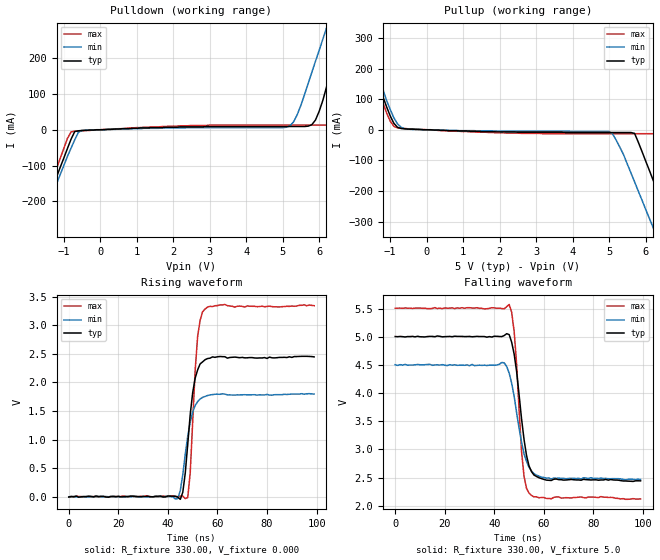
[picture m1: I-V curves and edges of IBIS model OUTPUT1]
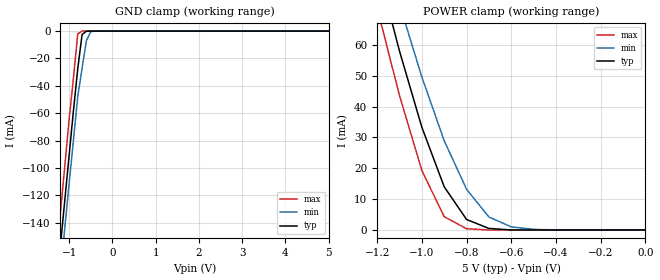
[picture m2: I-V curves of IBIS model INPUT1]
| IBIS file 8581nb5v.ibs
[IBIS ver]   2.1
[File name]   8581nb5v.ibs
[File Rev]   1.0
[Date]   July 4, 2003
[Source]   This file orginated at SEIKO EPSON QD Div.
   This file is for 5.0V CMOS parts.
[Copyright]   Copyright SEIKO EPSON Corp. 2003
|   Component RX-8581NB
[Component]   RX-8581NB
[Manufacturer]   SEIKO EPSON
[Package]
| variable   typ   min   max
R_pkg   87m   NA   NA
L_pkg   10nH   NA   NA
C_pkg   206fF   NA   NA
[Pin]  signal_name   model_name   R_pin   L_pin   C_pin
|1   /INT
2   GND   GND
|3   (VDD)
|4   NC
|5   SDA
|6   SCL
7   FOUT   OUTPUT1
8   VDD   POWER
9   FOE   INPUT1
| Models and submodels in the file (2): OUTPUT1 (Output), INPUT1 (Input)
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|10   NC
|11   NC
|12   NC
|13   NC
|14   NC
|15   NC
|16   NC
|17   NC
|18   NC
|19   NC
|20   NC
|21   NC
|22   NC
|   Model OUTPUT
[Model]   OUTPUT1
Model_type   Output
Polarity   Non-Inverting
Enable   Active-High
Vmeas =   1.50V
C_comp   1.69pF   1.32pF   1.96pF
[Temperature Range]   25.00   85.00   -40.000
[Voltage Range]   5.0V   4.5V   5.5V
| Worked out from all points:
|   slope of the pulldown table from 0 to 0.75 V, typ, clamps not added: 250 ohm
|   slope of the pullup table from 0 to 0.75 V, typ, clamps not added: 250 ohm
|   rising waveform, R_fixture 330.00, V_fixture 0.000: 20-80 % time 3.39ns typ, 3.85ns min, 2.5ns max; typ from -0.005 V to 2.45 V
|   falling waveform, R_fixture 330.00, V_fixture 5.0: 20-80 % time 4.13ns typ, 5.01ns min, 2.91ns max; typ from 5.01 V to 2.44 V
[Pulldown]
| voltage   I(typ)   I(min)   I(max)
-5V       -1.155A    -1.128A    -1.18A
-2V       -348mA     -357mA     -334mA
-1.5V     -213mA     -228mA     -193mA
-800mV    -26mA      -51mA      -6mA
-500mV    -2mA       -2mA       -3mA
5.2V      9mA        11mA       13mA
5.9V      27mA       191mA      13mA
6.3V      155mA      313mA      13mA
6.7V      303mA      436mA      97mA
7V        414mA      528mA      200mA
7.5V      598mA      681mA      372mA
10V       1.522A     1.447A     1.231A
[Pullup]
| voltage   I(typ)   I(min)   I(max)
-5V       1.467A     1.5A       1.488A
-2V       393mA      420mA      378mA
-1.5V     214mA      240mA      193mA
-1V       45mA       66mA       28mA
-700mV    4mA        8mA        5mA
5V        -9mA       -6mA       -13mA
5.3V      -9mA       -58mA      -13mA
5.7V      -12mA      -170mA     -13mA
6.3V      -192mA     -347mA     -15mA
6.8V      -345mA     -494mA     -156mA
7.5V      -558mA     -700mA     -354mA
10V       -1.321A    -1.435A    -1.062A
[Ramp]
| variable   typ   min   max
dV/dt_r 1.08/2.1n   0.88/2.7n   0.74/1n
dV/dt_f 0.6/1.8n   0.67/2.7n   1.04/1.7n
R_load = 330.00
[Rising Waveform]
R_fixture = 330.00
V_fixture = 0.000
| time   V(typ)   V(min)   V(max)
0s        -5mV       -1mV       -3mV
44ns      -8mV       -31mV      1mV
46ns      78mV       388mV      12mV
48ns      920mV      1.061V     -14mV
49ns      1.439V     1.304V     420mV
51ns      2.076V     1.597V     2.218V
52ns      2.221V     1.664V     2.81V
54ns      2.36V      1.739V     3.238V
63ns      2.45V      1.796V     3.364V
99ns      2.447V     1.796V     3.343V
[Falling Waveform]
R_fixture = 330.00
V_fixture = 5.0
V_fixture_min = 4.5
V_fixture_max = 5.5
| time   V(typ)   V(min)   V(max)
0s        5.006V     4.505V     5.509V
43ns      5.005V     4.545V     5.504V
46ns      5.04V      4.356V     5.575V
48ns      4.694V     3.945V     5.095V
49ns      4.383V     3.653V     4.514V
51ns      3.539V     3.127V     2.957V
52ns      3.174V     2.921V     2.521V
54ns      2.709V     2.683V     2.226V
61ns      2.456V     2.492V     2.131V
99ns      2.443V     2.468V     2.122V
|   Model INPUT1
[Model]   INPUT1
Model_type   Input
Polarity   Non-Inverting
Vinl =   1.00V
Vinh =   2.20V
C_comp   0.80pF   0.60pF   1.00pF
[Temperature Range]   25.00   85.00   -40.00
[Voltage Range]   5.0V   4.5V   5.50V
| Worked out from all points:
|   GND clamp passes 1 mA (typ) near -0.64 V on its own axis
|   POWER clamp passes 1 mA (typ) near -0.72 V on its own axis
[GND_clamp]
| voltage   I(typ)   I(min)   I(max)
-5V       -1.403A    -1.393A    -1.425A
-1.3V     -189.4mA   -207.9mA   -166.7mA
-1.2V     -156.6mA   -175.9mA   -132.7mA
-1.1V     -123.8mA   -143.9mA   -98.7mA
-1V       -91mA      -111.8mA   -64.7mA
-900mV    -58.2mA    -79.8mA    -34.4mA
-800mV    -27.5mA    -47.8mA    -2.1mA
-700mV    -2.5mA     -27.1mA    0A
-600mV    -100uA     -7mA       0A
-500mV    0A         -500uA     0A
-400mV    0A         0A         0A
5V        0A         0A         0A
[POWER_clamp]
| voltage   I(typ)   I(min)   I(max)
-5V       1.121A     1.157A     1.136A
-1.2V     85.8mA     98.5mA     72mA
-1.1V     58mA       73.2mA     43.6mA
-1V       33.3mA     49.6mA     19.3mA
-900mV    14mA       28.9mA     4.3mA
-800mV    3.4mA      13.2mA     400uA
-700mV    500uA      4.2mA      0A
-600mV    0A         1mA        0A
-500mV    0A         200uA      0A
-400mV    0A         0A         0A
0V        0A         0A         0A
